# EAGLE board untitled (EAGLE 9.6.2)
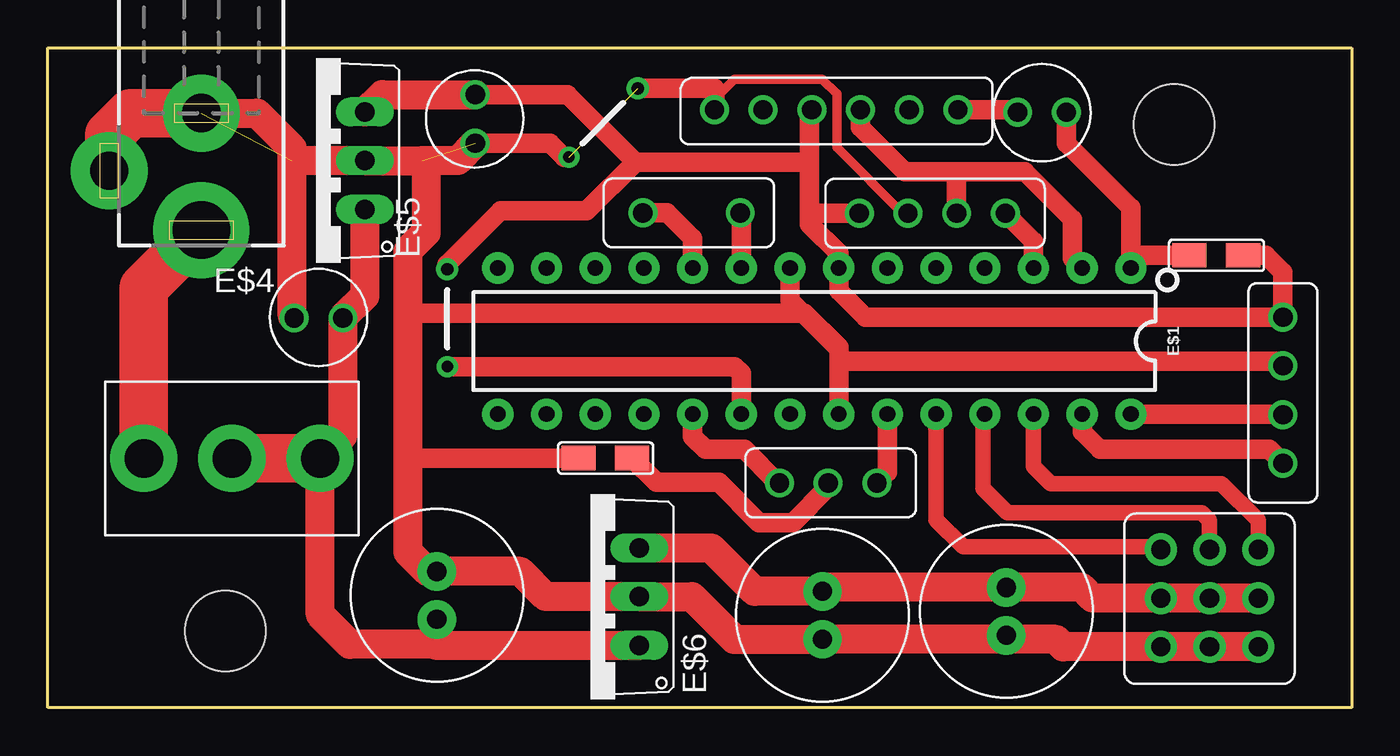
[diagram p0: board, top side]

Size 68 x 34.4 mm. Coordinates in mm from the lower left corner, seen from the top.
Outline: 0,0 0,34.4 68,34.4 68,0 0,0
Copper layers (1*16): Top 0.035mm / dielectric 1.5mm / Bottom 0.035mm
Design rules "default": minimum track width 6mil, minimum drill 0.35mm, track to track 6mil, track to pad 6mil, pad to pad 6mil, via to via 6mil, smd to smd 6mil, copper to edge 40mil, drill to drill 6mil, minimum pad ring 10mil, minimum via ring 8mil, stop-mask expansion 4mil, vias tented up to drill 0mil, thermal gap 10mil
Holes 4.2 mm at 9.25,4 58.75,30.4

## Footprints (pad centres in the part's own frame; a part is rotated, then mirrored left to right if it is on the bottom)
DIP28 = drill 0.813 pad 1.626: 1 -16.51,-3.81; 2 -13.97,-3.81; 3 -11.43,-3.81; 4 -8.89,-3.81; 5 -6.35,-3.81; 6 -3.81,-3.81; 7 -1.27,-3.81; 8 1.27,-3.81; 9 3.81,-3.81; 10 6.35,-3.81; 11 8.89,-3.81; 12 11.43,-3.81; 13 13.97,-3.81; 14 16.51,-3.81; 15 16.51,3.81; 16 13.97,3.81; 17 11.43,3.81; 18 8.89,3.81; 19 6.35,3.81; 20 3.81,3.81; 21 1.27,3.81; 22 -1.27,3.81; 23 -3.81,3.81; 24 -6.35,3.81; 25 -8.89,3.81; 26 -11.43,3.81; 27 -13.97,3.81; 28 -16.51,3.81
INTERRUPTOR = drill 2 pad 3.5: P$1 2,4; P$2 6.6,4; P$3 11.2,4
XTAL_16_MHZ = drill 1: 1 1.27,1.3; 3 6.35,1.3
DCJ0202 = drill 3 pad 5: 1 0,3.1 | drill 2 pad 4: 2 4.8,0; 3 0,-3
TO220V = drill 1.016 long: 1 -2.54,-2.54; 2 0,-2.54; 3 2.54,-2.54
CONDENSADOR = drill 1: 1 1.27,1.3; 2 3.81,1.3
CONDENSADOR_8MM_DIAMETRO = drill 1 pad 2: P$1 0,0; P$2 0,2.5
CONECTOR_3X3_PINES = drill 1 pad 1.676: 1 1.27,1.3; 2 3.81,1.3; 3 6.35,1.3; 4 3.81,3.84; 5 1.27,3.84; 6 6.35,3.84; 7 1.27,6.38; 8 3.81,6.38; 9 6.35,6.38
CONECTOR_4_PINES = drill 1: 1 1.27,1.3; 2 3.81,1.3; 3 6.35,1.3; 4 8.89,1.3
0805 = smd 1.27 x 1.778: 1 0.635,0.889; 2 0.635,3.683
CONECTOR_6_PINES = drill 1: 1 1.27,1.3; 2 3.81,1.3; 3 6.35,1.3; 4 8.89,1.3; 5 11.43,1.3; 6 13.97,1.3
CONECTOR_3_PINES = drill 1: 1 1.27,1.3; 2 3.81,1.3; 3 6.35,1.3
PUENTE_0.2INCH = drill 0.6: P$1 0,0 | drill 0.65: P$2 5.08,0

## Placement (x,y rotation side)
E$1  [DIP28]  39.98,19.12 180 top
E$2  [INTERRUPTOR]  3,9 0 top
E$3  [XTAL_16_MHZ]  37.38,27.1 180 top
E$4  [DCJ0202]  8,28 180 top
E$5  [TO220V]  13.99,28.52 90 top
E$6  [TO220V]  28.3,5.79 90 top
E$7  [CONDENSADOR]  20.99,33.24 270 top
E$8  [CONDENSADOR_8MM_DIAMETRO]  40.4,3.56 0 top
E$9  [CONDENSADOR_8MM_DIAMETRO]  49.99,3.77 0 top
E$10  [CONDENSADOR_8MM_DIAMETRO]  20.29,7.1 180 top
E$11  [CONECTOR_3X3_PINES]  56.78,1.87 0 top
E$12  [CONECTOR_4_PINES]  63.12,21.63 270 top
E$14  [0805]  31.36,12.38 90 top
E$15  [0805]  63.23,22.95 90 top
E$16  [CONECTOR_4_PINES]  41.05,24.48 0 top
E$17  [CONECTOR_6_PINES]  33.49,29.88 0 top
E$18  [CONECTOR_3_PINES]  36.89,10.42 0 top
E$19  [CONDENSADOR]  49.31,29.75 0 top
E$20  [CONDENSADOR]  16.66,21.62 180 top
E$21  [PUENTE_0.2INCH]  27.18,28.7 45 top
E$22  [PUENTE_0.2INCH]  20.83,17.78 90 top

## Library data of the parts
E$1 = SparkFun-IC-Microcontroller
E$2 E$3 E$7 E$11 E$12 E$14-E$20 = ALT_F4_LIB
E$4 = con-jack
E$5 E$6 = DC_LOAD_AU
E$8-E$10 E$21 E$22 = Mi_Librería

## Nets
S$1: E$2.P$1 E$4.1
S$2: E$6.3 E$8.P$2 E$9.P$2 E$11.4 E$11.5 E$11.6
S$3: E$1.26 E$11.9
S$4: E$1.10 E$3.3
S$5: E$1.25 E$11.8
S$6: E$2.P$2 E$2.P$3 E$5.1 E$6.1 E$10.P$2 E$20.1
S$7: E$1.9 E$3.1
S$8: E$1.24 E$11.7
S$9: E$1.27 E$12.4
S$10: E$1.28 E$12.3
S$11: E$1.8 E$1.22 E$4.2 E$4.3 E$5.2 E$6.2 E$7.2 E$8.P$1 E$9.P$1 E$10.P$1 E$11.1 E$11.2 E$11.3 E$12.2 E$14.2 E$16.2 E$17.1 E$20.2 E$21.P$1 E$21.P$2
S$12: E$1.7 E$5.3 E$7.1 E$12.1 E$15.1 E$16.1 E$17.3 E$22.P$2
S$13: E$1.3 E$16.4
S$14: E$1.2 E$16.3 E$17.4
S$15: E$17.6 E$19.1
S$16: E$1.1 E$15.2 E$19.2
S$17: E$1.20 E$22.P$1
S$18: E$1.23 E$18.3
S$19: E$1.19 E$18.1
S$20: E$14.1 E$18.2

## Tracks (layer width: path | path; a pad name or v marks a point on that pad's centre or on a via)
S$1
  Top 2.54: E$4.1 5,21.9 E$2.P$1
S$2
  Top 1.524: E$11.6 E$11.4 E$11.5 54.49,5.71 53.93,6.27 E$9.P$2 40.6,6.27 E$8.P$2 36.86,6.06 34.6,8.32 E$6.3
S$3
  Top 0.813: E$1.26 51.41,12.6 52.32,11.68 61.21,11.68 63.13,9.77 E$11.9
S$4
  Top 1.016: E$3.3 32.3,25.8 33.63,24.47 E$1.10
S$5
  Top 0.813: 48.77,15.21 48.77,11.43 50.04,10.16 60.2,10.16 60.59,9.77 E$11.8
  Top 1.016: E$1.25 48.77,15.21
S$6
  Top 1.524: E$5.1 16.53,21.46 E$20.1 15.38,14.19 E$2.P$3 14.2,4.85 15.75,3.3 20.29,3.3 E$10.P$2 20.29,3.25 E$6.1
  Top 2.54: E$2.P$3 E$2.P$2
S$7
  Top 1.016: E$1.9 36.17,25.74 E$3.1
S$8
  Top 0.813: E$1.24 46.33,9.81 47.75,8.38 57.92,8.38 E$11.7
S$9
  Top 1.016: E$1.27 53.95,14.38 54.86,13.46 63.7,13.46 E$12.4
S$10
  Top 1.016: E$1.28 64.4,15.31 E$12.3
S$11  (3 unrouted)
  Top 0.508: E$17.1 35.05,31.46 35.05,32 35.81,32.77 40.39,32.77 41.15,32 41.15,29.21 44.58,25.78 E$16.2
  Top 1.016: E$17.1 34.76,32.29 E$21.P$2 | E$21.P$1 26.92,28.7 26.2,29.43 E$7.2 | E$1.22 41.25,18.08 64.17,18.08 E$12.2 | E$1.22 41.25,18.8 39.47,20.57 18.77,20.57 | E$1.8 38.71,21.24 41.25,18.7 E$1.22 | E$14.2 18.96,13.02 18.77,13.21
  Top 1.524: E$7.2 21.39,28.52 19.73,28.52 19.73,24.78 18.77,23.82 18.77,20.57 18.77,13.21 18.77,8.12 19.78,7.1 E$10.P$1 24.65,7.1 25.96,5.79 E$6.2 33.59,5.79 35.81,3.56 E$8.P$1 49.78,3.56 E$9.P$1 50.2,3.56 52.58,3.56 52.96,3.17 E$11.1 E$11.2 E$11.3 | E$20.2 12.75,20.41 12.75,29.16 10.91,31 E$4.3 | 19.53,28.52 E$5.2 12.75,28.52
  Top 2.54: E$4.3 4.33,31 3.2,29.87 E$4.2
S$12
  Top 1.016: 39.72,28.45 39.72,25.91 | 39.72,25.91 39.72,25.21 41.25,23.69 E$1.7 41.25,21.74 42.63,20.36 E$12.1 64.42,22.7 63.53,23.59 E$15.1 | 39.72,28.45 30.64,28.45 | 30.64,28.45 27.12,31.97 E$7.1 | E$16.1 39.85,25.78 39.72,25.91 | E$17.3 39.72,31.06 39.72,28.45 | E$22.P$2 20.83,23.11 23.62,25.91 28.1,25.91 30.64,28.45
  Top 1.524: E$5.3 17.43,31.97 E$7.1
S$13
  Top 1.016: E$16.4 51.41,24.31 E$1.3
S$14
  Top 1.016: E$1.2 53.44,23.43 53.44,25.47 50.97,27.94 47.4,27.94 | 47.4,27.94 E$16.3 | 47.4,27.94 44.7,27.94 42.38,30.26 E$17.4
S$15
  Top 1.016: E$17.6 50.46,31.18 E$19.1
S$16
  Top 1.016: E$19.2 53.12,29.43 56.49,26.06 E$1.1 56.49,23.07 57,23.59 E$15.2
S$17
  Top 1.016: E$1.20 36.17,17.43 35.81,17.78 E$22.P$1
S$18
  Top 1.016: E$1.23 43.79,12.27 E$18.3
S$19
  Top 1.016: E$18.1 38.07,11.72 36.32,13.46 34.29,13.46 33.63,14.12 E$1.19
S$20
  Top 1.016: E$14.1 31.74,11.74 34.99,11.74 37.08,9.65 38.86,9.65 40.7,11.49 E$18.2

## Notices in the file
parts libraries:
SparkFun-IC-Microcontroller: Licensing: Creative Commons ShareAlike 4.0 International - https://creativecommons.org/licenses/by-sa/4.0
